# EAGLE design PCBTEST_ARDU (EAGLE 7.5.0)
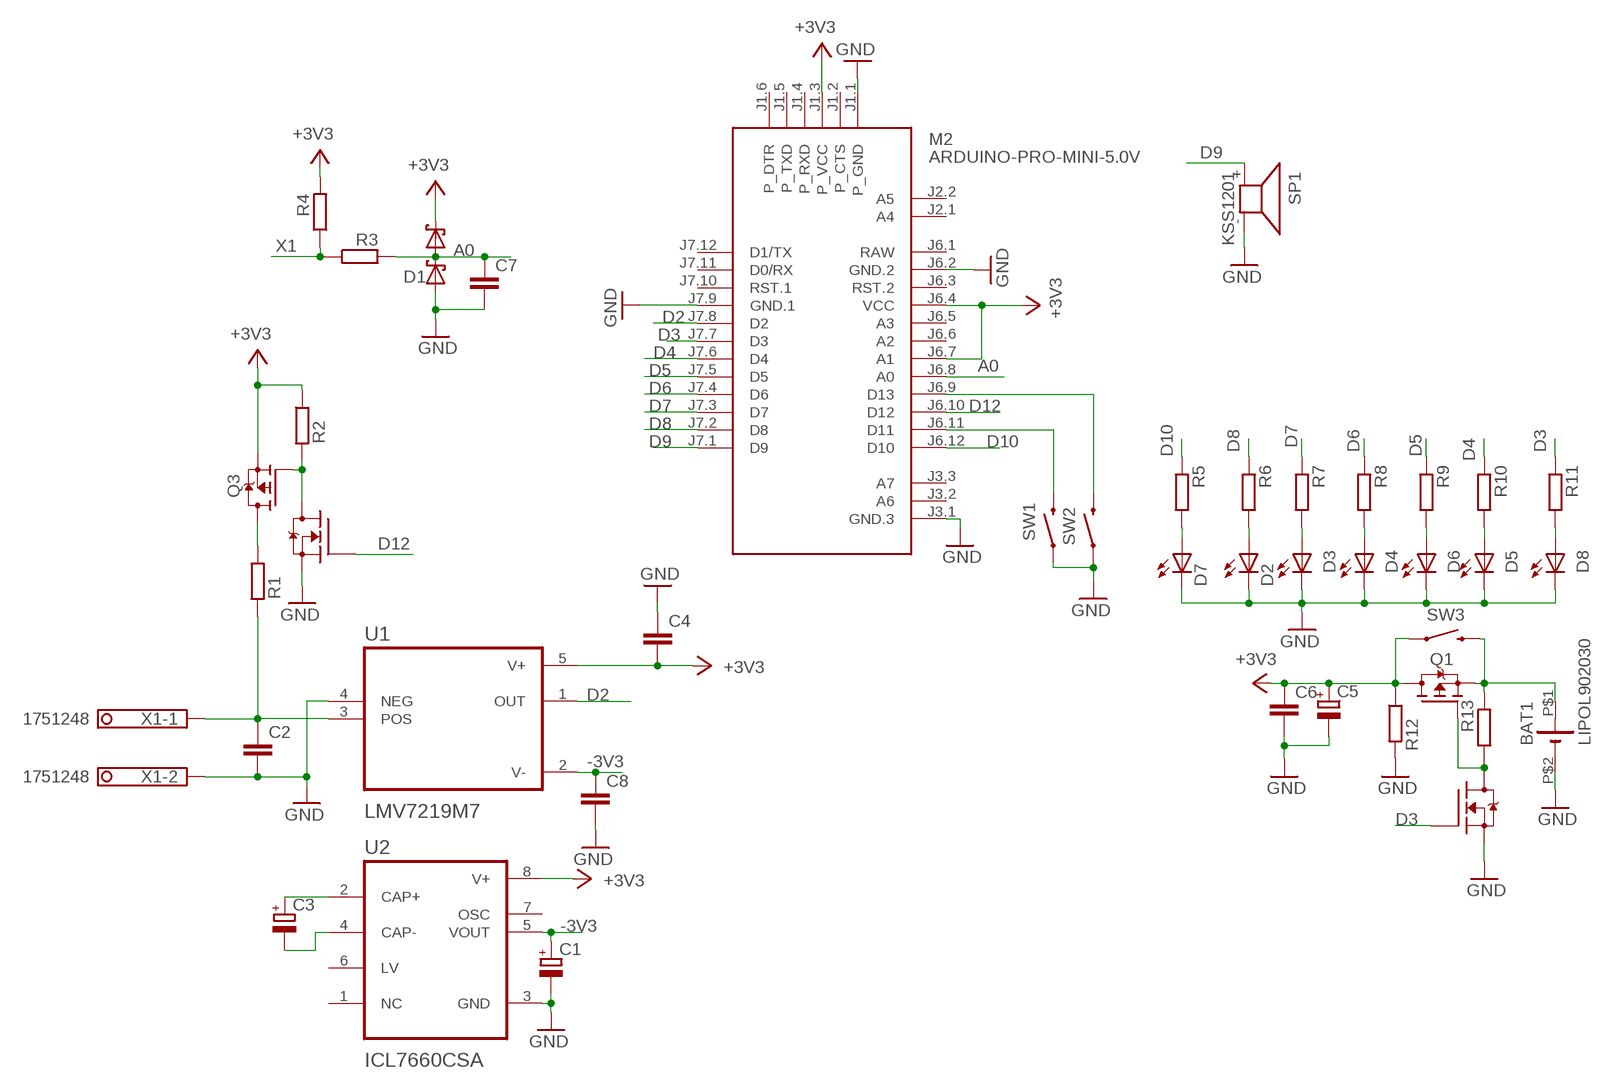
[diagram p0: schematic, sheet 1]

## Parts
BAT1  LIPOL902030  [LIPOL902030]
C1  CPOL-EUSMCA  [SMC_A]
C2  C-EUC1206  [C1206]
C3  CPOL-EUSMCA  [SMC_A]
C4  C-EUC0603  [C0603]
C5  CPOL-EUSMCA  [SMC_A]
C6  C-EUC0603  [C0603]
C7  C-EUC0603  [C0603]
C8  C-EUC0603  [C0603]
D1  BAT54S  [SOT23]
D2  LEDCHIPLED_0805  [CHIPLED_0805]
D3  LEDCHIPLED_0805  [CHIPLED_0805]
D4  LEDCHIPLED_0805  [CHIPLED_0805]
D5  LEDCHIPLED_0805  [CHIPLED_0805]
D6  LEDCHIPLED_0805  [CHIPLED_0805]
D7  LEDCHIPLED_0805  [CHIPLED_0805]
D8  LEDCHIPLED_0805  [CHIPLED_0805]
M2  ARDUINO-PRO-MINI-5.0V  [ARDUINO-PRO-MINI]
Q1  STR2P3LLH6  [SOT23]
Q2  ZVN3310F  [SOT23]
Q3  STR2P3LLH6  [SOT23]
Q5  ZVN3310F  [SOT23]
R1  R-EU_R0603  [R0603]
R2  R-EU_R0603  [R0603]
R3  R-EU_R0603  [R0603]
R4  R-EU_R0603  [R0603]
R5  R-EU_R0603  [R0603]
R6  R-EU_R0603  [R0603]
R7  R-EU_R0603  [R0603]
R8  R-EU_R0603  [R0603]
R9  R-EU_R0603  [R0603]
R10  R-EU_R0603  [R0603]
R11  R-EU_R0603  [R0603]
R12  R-EU_R0603  [R0603]
R13  R-EU_R0603  [R0603]
SP1  KSS1201  [KSS1201]
SW1  SWITCH-MOMENTARY-2SMD  [TACTILE-SWITCH-SMD]
SW2  SWITCH-MOMENTARY-2SMD  [TACTILE-SWITCH-SMD]
SW3  SWITCH-MOMENTARY-2SMD  [TACTILE-SWITCH-SMD]
U1  LMV7219M7  [SOT65P210X110-5N]
U2  ICL7660CSA  [SOIC127P600X175-8N]
X1  1751248  [1751248]

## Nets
+3V3: C4.2 C5.+ C6.1 D1.2(C2) M2.J1.3(P_VCC) M2.J6.4(VCC) M2.J6.7(A1) Q1.1(D) Q3.3(S) R2.1 R4.2 R12.1 SW3.1 U1.5(V+) U2.8(V+)
-3V3: C1.+ C8.1 U1.2(V-) U2.5(VOUT)
A0: C7.1 D1.3(C1A2) M2.J6.8(A0) R3.2
D2: M2.J7.8(D2) U1.1(OUT)
D3: M2.J7.7(D3) Q5.2(G) R11.1
D4: M2.J7.6(D4) R10.1
D5: M2.J7.5(D5) R9.1
D6: M2.J7.4(D6) R8.1
D7: M2.J7.3(D7) R7.1
D8: M2.J7.2(D8) R6.1
D9: M2.J7.1(D9) SP1.+
D10: M2.J6.12(D10) R5.1
D12: M2.J6.10(D12) Q2.2(G)
GND: BAT1.P$2(-) C1.- C2.2 C4.1 C5.- C6.2 C7.2 C8.2 D1.1(A1) D2.C D3.C D4.C D5.C D6.C D7.C D8.C M2.J1.1(P_GND) M2.J3.1(GND.3) M2.J6.2(GND.2) M2.J7.9(GND.1) Q2.3(S) Q5.3(S) R12.2 SP1.- SW1.1 SW2.1 U1.4(NEG) U2.3(GND) X1.2
N$1: C3.+ U2.2(CAP+)
N$2: C3.- U2.4(CAP-)
N$3: C2.1 R1.2 U1.3(POS) X1.1
N$4: Q2.1(D) Q3.2(G) R2.2
N$5: M2.J6.11(D11) SW1.3
N$6: Q3.1(D) R1.1
N$7: M2.J6.9(D13) SW2.3
N$11: D3.A R7.2
N$12: D2.A R6.2
N$13: D7.A R5.2
N$15: BAT1.P$1(+) Q1.3(S) R13.2 SW3.3
N$16: D4.A R8.2
N$17: Q1.2(G) Q5.1(D) R13.1
N$19: D6.A R9.2
N$21: D5.A R10.2
N$23: D8.A R11.2
X1: R3.1 R4.1
Unconnected: M2.J1.2(P_CTS) M2.J1.4(P_RXD) M2.J1.5(P_TXD) M2.J1.6(P_DTR) M2.J2.1(A4) M2.J2.2(A5) M2.J3.2(A6) M2.J3.3(A7) M2.J6.3(RST.2) M2.J6.5(A3) M2.J6.6(A2) M2.J7.10(RST.1) M2.J7.11(D0/RX) M2.J7.12(D1/TX) U2.1(NC) U2.6(LV) U2.7(OSC)

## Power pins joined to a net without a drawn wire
RAW: M2.J6.1(RAW)

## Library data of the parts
BAT1 = battery:LIPOL902030
C1 C3 C5 = rcl:CPOL-EU: POLARIZED CAPACITOR, European symbol
C2 C4 C6-C8 = rcl:C-EU: CAPACITOR, European symbol
D1 = diode:BAT54S: Schottky Diodes Pin connection corrected 2011-05-04 Source: Fairchild .. BAT54.pdf
D2-D8 = led:LED: LED
M2 = diy-modules:ARDUINO-PRO-MINI-*: Arduino Pro Mini and compatible devices More details available here: https://www.arduino.cc/en/Main/ArduinoBoardProMini Click here to find device on ebay.com
Q1 Q3 = transistor-fet:STR2P3LLH6
Q2 Q5 = transistor-fet:ZVN3310F
R1-R13 = rcl:R-EU_: RESISTOR, European symbol
SP1 = buzzer:KSS1201: SPEAKER; OC_FARNELL: unknown; OC_NEWARK: unknown
SW1-SW3 = SparkFun-Electromechanical:SWITCH-MOMENTARY-2: Various NO switches- pushbuttons, reed, etc; PROD_ID: SWCH-08247
U1 = LMV7219M7:LMV7219M7: Check availability; AVAILABILITY: In Stock; CHECK_PRICES: https://www.snapeda.com/parts/LMV7219M7/Texas+Instruments/view-part/?ref=eda; DESCRIPTION: 7 nsec, 2.7V to 5V Comparator with Rail-to- Rail Output; MF: Texas Instruments; MP: LMV7219M7; PACKAGE: SC70-5 Texas Instruments; PRICE: None; SNAPEDA_LINK: https://www.snapeda.com/parts/LMV7219M7/Texas+Instruments/view-part/?ref=snap
U2 = ICL7660CSA:ICL7660CSA: Check availability; AVAILABILITY: In Stock; CHECK_PRICES: https://www.snapeda.com/parts/ICL7660CSA/Analog+Devices/view-part/?ref=eda; DESCRIPTION: Charge Pump Switching Regulator IC Positive or Negative Fixed -Vin, nVin, Vin/2 1 Output 20mA 8-SOIC (0.154, 3.90mm Width); MF: Analog Devices; MP: ICL7660CSA; PACKAGE: SOIC-8 Maxim; PRICE: None; SNAPEDA_LINK: https://www.snapeda.com/parts/ICL7660CSA/Analog+Devices/view-part/?ref=snap
X1 = con-phoenix-350:1751248: MKDS 1/ 2-3,5 Printklemme; OC_FARNELL: unknown; OC_NEWARK: unknown

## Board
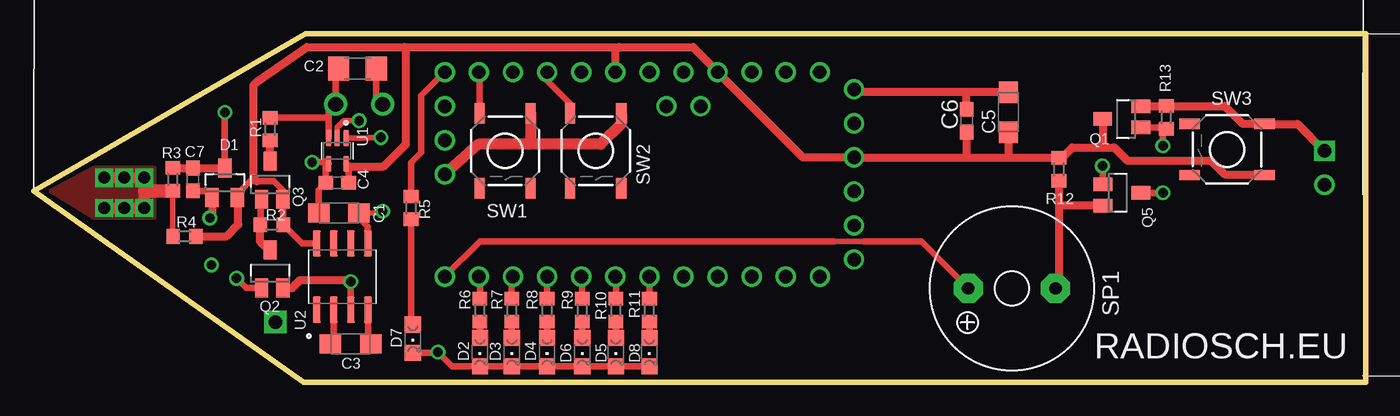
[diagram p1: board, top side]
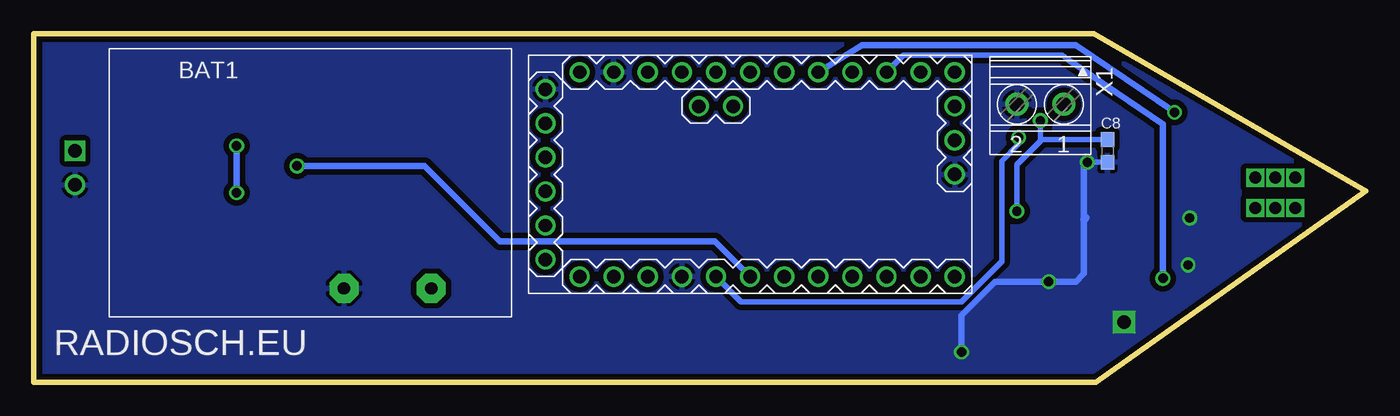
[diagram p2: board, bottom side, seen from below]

Size 99.25 x 26 mm. Coordinates in mm from the lower left corner, seen from the top.
Outline: 0,14.25 20.25,26 99.25,26 99.25,0 20.12,0 0,14.25
Copper layers (1*16): Top 0.035mm / dielectric 1.5mm / Bottom 0.035mm
Design rules "default *": minimum track width 10mil, minimum drill 20mil, track to track 6mil, track to pad 6mil, pad to pad 6mil, via to via 6mil, smd to smd 6mil, copper to edge 6mil, drill to drill 6mil, minimum pad ring 10mil, minimum via ring 8mil, stop-mask expansion 4mil, vias tented up to drill 20mil, thermal gap 10mil

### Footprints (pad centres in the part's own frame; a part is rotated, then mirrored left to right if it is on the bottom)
LIPOL902030 = drill 1 square: P$1 -2.54,-7.62 | drill 1: P$2 -2.54,-10.16
SMC_A = smd 1.6 x 1.4: + -1.5,0; - 1.5,0
C1206 = smd 1.6 x 1.8: 1 -1.4,0; 2 1.4,0
C0603 = smd 1.1 x 1: 1 -0.85,0; 2 0.85,0
SOT23 = smd 1 x 1.4: 1 -0.95,-1.1; 2 0.95,-1.1; 3 0,1.1
CHIPLED_0805 = smd 1.2 x 1.2: A 0,-1.05; C 0,1.05
ARDUINO-PRO-MINI = drill 1: J1.1 -15.24,6.35; J1.2 -15.24,3.81; J1.3 -15.24,1.27; J1.4 -15.24,-1.27; J1.5 -15.24,-3.81; J1.6 -15.24,-6.35; J2.1 -1.27,5.08; J2.2 -3.81,5.08; J3.1 15.24,0; J3.2 15.24,2.54; J3.3 15.24,5.08; J6.1 -12.7,7.62; J6.2 -10.16,7.62; J6.3 -7.62,7.62; J6.4 -5.08,7.62; J6.5 -2.54,7.62; J6.6 0,7.62; J6.7 2.54,7.62; J6.8 5.08,7.62; J6.9 7.62,7.62; J6.10 10.16,7.62; J6.11 12.7,7.62; J6.12 15.24,7.62; J7.1 15.24,-7.62; J7.2 12.7,-7.62; J7.3 10.16,-7.62; J7.4 7.62,-7.62; J7.5 5.08,-7.62; J7.6 2.54,-7.62; J7.7 0,-7.62; J7.8 -2.54,-7.62; J7.9 -5.08,-7.62; J7.10 -7.62,-7.62; J7.11 -10.16,-7.62; J7.12 -12.7,-7.62
SOT23' = smd 1 x 1.4: 1 0,1.735; 2 -0.632,-1.1; 3 0.95,-1.1
R0603 = smd 1 x 1.1: 1 -0.85,0; 2 0.85,0
KSS1201 = drill 0.914 pad 2.159 octagon: + 3.251,0; - -3.251,0
TACTILE-SWITCH-SMD = smd 1.524 x 0.762: 1 -2.794,1.905; 2 2.794,1.905; 3 -2.794,-1.905; 4 2.794,-1.905
SOT65P210X110-5N = smd 1.19 x 0.4: 1 -0.96,0.65; 2 -0.96,0; 3 -0.96,-0.65; 4 0.96,-0.65; 5 0.96,0.65
SOIC127P600X175-8N = smd 1.97 x 0.59: 1 -2.475,1.905; 2 -2.475,0.635; 3 -2.475,-0.635; 4 -2.475,-1.905; 5 2.475,-1.905; 6 2.475,-0.635; 7 2.475,0.635; 8 2.475,1.905
1751248 = drill 1.1 pad 1.7: 1 -1.75,-0.1; 2 1.75,-0.1

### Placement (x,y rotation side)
BAT1  93.62,24.88 0 bottom
C1  22.75,12.62 180 top
C2  24.12,23.38 0 top
C3  23.62,2.88 0 top
C4  22.62,14.88 0 top
C5  72.62,20.12 90 top
C6  69.5,19.5 90 top
C7  11.88,15.12 270 top
C8  19.25,17.25 270 bottom
D1  14.25,14.88 0 top
D2  33.25,2.25 180 top
D3  35.62,2.25 180 top
D4  38.25,2.25 180 top
D5  43.38,2.25 180 top
D6  40.88,2.25 180 top
D7  28.25,3.25 180 top
D8  45.88,2.25 180 top
M2  45.88,15.5 0 bottom
Q1  STR2P3LLH6  [SOT23']  81.38,19.62 90 top
Q2  ZVN3310F  [SOT23']  17.62,8.12 0 top
Q3  STR2P3LLH6  [SOT23']  17.62,14.75 0 top
Q5  ZVN3310F  [SOT23']  80.75,14.12 270 top
R1  17.62,18.88 90 top
R2  17.75,11.75 180 top
R3  10.38,15.12 90 top
R4  11.25,10.88 0 top
R5  28.12,13 270 top
R6  33.25,5.38 270 top
R7  35.62,5.38 270 top
R8  38.25,5.38 270 top
R9  40.88,5.38 270 top
R10  43.38,5.38 270 top
R11  45.88,5.38 270 top
R12  76.38,15.88 270 top
R13  84.38,19.75 90 top
SP1  72.88,7 180 top
SW1  35.12,17.25 270 top
SW2  41.88,17.25 270 top
SW3  88.9,17.36 180 top
U1  22.62,17.25 270 top
U2  23,7.88 90 top
X1  24.25,20.62 180 bottom

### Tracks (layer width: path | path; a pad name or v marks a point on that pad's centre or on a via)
+3V3
  Top 0.5: 15.25,12.88 15.25,13.72 | D1.2 15.2,14.07 16.12,15 16.62,15 17.88,15 18.57,14.3 Q3.3 18.6,13.62 R2.1 20,10.35 U2.8 | C4.2 23.48,16.09 U1.5
  Top 0.61: 16.62,15 16.38,15.25 16.38,22.12 16.62,22.38 20.38,25 27.62,25 | 27.62,25 43.62,25 | 43.62,25 49.12,25 50.95,23.17 M2.J6.4 57.3,16.77 M2.J1.3 69.62,16.77 | M2.J6.7 43.34,24.71 43.62,25 | R4.2 14.38,10.88 15.25,11.75 15.25,13.72 D1.2 | 23.48,16.09 26.09,16.09 27.75,17.75 27.75,24.88 27.62,25 | 69.62,16.77 72.5,16.77 | 72.5,16.77 76.33,16.77 R12.1 76.6,16.73 77.38,17.5 79.75,17.5 | 79.75,17.5 80.5,17.5 81.5,16.5 87.75,16.5 88.75,15.5 91.65,15.5 SW3.1 | Q1.1 79.64,17.61 79.75,17.5 | C5.+ 72.62,16.89 72.5,16.77 | C6.1 69.5,16.89 69.62,16.77
-3V3  (via drill 0.7)
  Top 0.406: C1.+ 25.88,12.62 v26,12.75 | v24.25,19.5 23.12,19.5 22.62,19 U1.2
  Top 0.5: C1.+ 24.25,12.25 24.88,11.62 24.88,10.38 U2.5
  Bottom 0.406: 24.25,18 v24.25,19.5 | 24.25,18 26,16.25 v26,12.75 | C8.1 24.15,18.1 24.25,18
A0  (via drill 0.7)
  Top 0.5: D1.3 v14.25,20.12
  Top 0.61: R3.2 C7.1 D1.3
  Bottom 0.5: v14.25,20.12 21.62,25.12 37.54,25.12 M2.J6.8
D2  (via drill 0.7)
  Top 0.406: U1.1 24.96,18.21 25,18.25 v25.88,18.25
  Bottom 0.406: v25.88,18.25 25.88,17.75 27.12,16.5 27.12,9 30.12,6 46.53,6 M2.J7.8
D3  (via drill 0.7)
  Top 0.5: R11.1 M2.J7.7 | Q5.2 79.65,16.1 v79.62,16.12
  Bottom 0.5: M2.J7.7 48.49,10.5 64.5,10.5 70.12,16.12 v79.62,16.12
D4
  Top 0.5: R10.1 43.38,7.84 M2.J7.6
D5
  Top 0.5: R9.1 40.88,7.8 M2.J7.5
D6
  Top 0.5: R8.1 M2.J7.4
D7
  Top 0.5: R7.1 35.62,7.79 M2.J7.3
D8
  Top 0.5: R6.1 33.25,7.8 M2.J7.2
D9
  Top 0.406: 61.88,10.5 59.62,10.5
  Top 0.5: 59.62,10.5 33.25,10.5 M2.J7.1 | 61.88,10.5 66.12,10.5 SP1.+
D10
  Top 0.5: R5.1 28.12,16.38 28.88,17.12 28.88,21.36 M2.J6.12
D12  (via drill 0.7)
  Top 0.5: Q2.2 15.85,7.03 v15.12,7.75
  Bottom 0.406: 22.12,24 22.62,24.38 34.46,24.38 M2.J6.10
  Bottom 0.5: v15.12,7.75 15.12,19.25 22.12,24
GND  (via drill 0.7, 1 pad 1.68)
  Top 0.5: C7.2 12.8,14.28 D1.1 | v20.75,16.4 21.86,16.4 U1.4 21.77,16.09 C4.1 21.25,14.35 C1.- | U2.3 v23.64,7.49 v23.62,7.5 | C2.2 25.52,21.2 X1.2 | D8.C D5.C D6.C D4.C D3.C D2.C 31.18,1.2 v30.12,2.25 30.07,2.2 D7.C
  Top 0.61: D1.1 13.3,12.43 v13.12,12.25 | Q2.3 19.27,7.03 19.88,7.62 23.5,7.62 v23.62,7.5 | R12.2 76.38,13.38 | 76.38,13.38 76.38,7.25 SP1.- | Q5.3 76.58,13.18 76.38,13.38 | C5.- 69.5,21.62 | 69.5,21.62 61.34,21.62 M2.J1.1 | C6.2 69.5,21.62
  Top 0.813: SW2.1 43.78,19.28 42.25,17.75 36.88,17.75 | 36.88,17.75 33.14,17.75 M2.J3.1 | SW1.1 37.03,17.91 36.88,17.75
  Bottom 0.406: C8.2 v20.75,16.4
  Bottom 0.5: v20.75,16.4 21,16.27 21,12.12 21,8.12 21.62,7.5 v23.62,7.5 27.62,7.5 30.12,5 v30.12,2.25
  Bottom 0.61: 20.88,12.25 21,12.12
  other vias: 13.25,8.75 18,4.5
  pour Bottom (isolate 0.406): 3,26.5 98.5,26.5 98.5,-1.12 3,-1.12
N$1
  Top 0.5: U2.2 22.36,3.12 C3.+
N$2
  Top 0.5: U2.4 24.91,3.1 C3.-
N$3
  Top 0.5: C2.1 22.5,23.15 X1.1 21.98,20.2 21.98,19.75 | U1.3 21.98,19.75 | R1.2 21.95,19.73 21.98,19.75
N$4
  Top 0.5: R2.2 16.9,13.56 Q3.2
  Top 0.61: Q2.1 17.52,9.86 16.88,10.5 16.88,11.72 R2.2
N$5
  Top 0.5: SW1.3 33.22,21.82 M2.J6.11
N$6
  Top 0.61: Q3.1 R1.1
N$7
  Top 0.5: M2.J6.9 38.26,22.49 40,20.75 40,20.07 SW2.3
N$11
  Top 0.5: D3.A R7.2
N$12
  Top 0.5: D2.A R6.2
N$13
  Top 0.5: R5.2 28.12,4.43 D7.A
N$15
  Top 0.61: Q1.3 84.35,20.57 R13.2 88.75,20.6 90.08,19.27 SW3.3 94.16,19.27 BAT1.P$1
N$16
  Top 0.5: D4.A R8.2
N$17  (via drill 0.7)
  Top 0.5: Q5.1 v84.12,14.12 | v84.12,17.62 84.12,18.65 R13.1 84.28,18.99 Q1.2
  Bottom 0.5: v84.12,14.12 v84.12,17.62
N$19
  Top 0.5: D6.A R9.2
N$21
  Top 0.5: D5.A R10.2
N$23
  Top 0.5: D8.A R11.2
X1  (via drill 0.9)
  Top 0.406: R3.1 10.38,11.85 R4.1
  Top 0.813: v5.25,15.25 v6.75,15.25 v8.25,15.25 8.25,14.25 | 8.25,14.25 v8.25,13 v6.75,13 v5.25,13 | 8.28,14.28 8.25,14.25
  Top 1.016: R3.1 8.28,14.28
  pour Top: 1.25,14.25 4.5,16 9,16 9,12.25 4.5,12.25

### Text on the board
tPlace: RADIOSCH.EU
bPlace: RADIOSCH.EU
